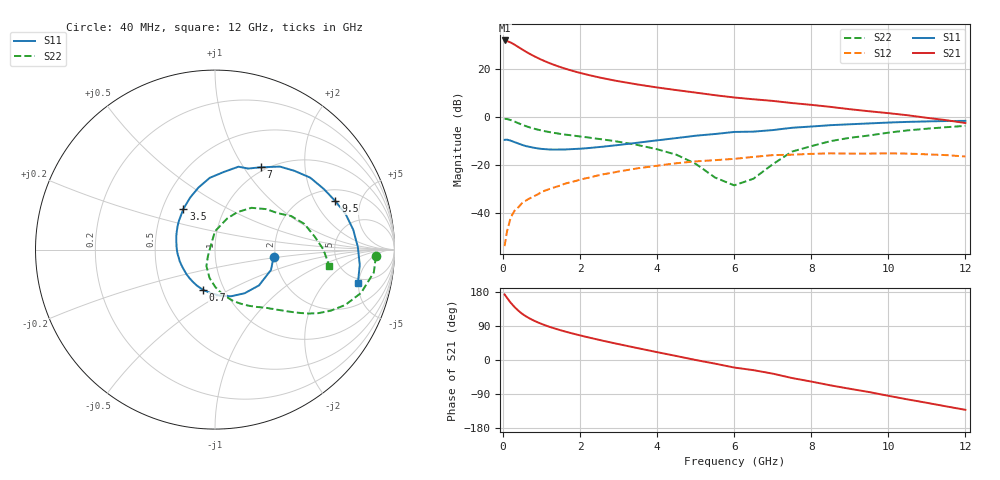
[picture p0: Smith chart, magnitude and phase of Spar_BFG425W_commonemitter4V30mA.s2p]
! Filename: 430bfg425.001
! BFG425W Field C1
! V1=8.371E-001V,V2=4.000E+000V, I1=3.822E-004A, I2=2.995E-002A
# GHz  S  MA  R 50
!  S11  S21  S12  S22
!Freq(GHz)  Mag  Ang  Mag  Ang  Mag  Ang  Mag  Ang
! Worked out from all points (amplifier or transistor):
!   44 points, 40 MHz to 12 GHz, reference 50 ohm
!   highest |S21| = 31.8 dB at 40 MHz (marker M1)
!   |S21| within 3 dB of that: start of sweep to 422.5 MHz
!   unconditionally stable (mu >= 1): start of sweep to 63.48 MHz; 1.129 GHz to end of sweep
!   at 700 MHz: K = 0.86, MSG = 30.0 dB, |S12| = -34.0 dB
!   at 2.4 GHz: K = 1.17, MAG = 18.2 dB, |S12| = -24.7 dB
!   at 12 GHz: K = 1.35, MAG = 3.4 dB, |S12| = -16.6 dB
!   S11 on the Smith chart (normalised r, x): 40 MHz: 1.96, -0.18; 700 MHz: 0.80, -0.38; 3.5 GHz: 0.64, +0.32; 7 GHz: 0.95, +1.20; 9.5 GHz: 2.63, +2.98; 12 GHz: 4.31, -4.89
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0.04  0.329 -7.3  38.74 173.0  0.002 47.2  0.897 -2.3
0.1  0.332 -19.9  37.77 164.5  0.004 70.2  0.894 -8.2
0.2  0.316 -39.1  35.07 150.8  0.008 70.2  0.849 -16.5
0.3  0.294 -55.8  31.55 139.6  0.011 68.4  0.789 -23.0
0.4  0.275 -71.0  28.15 129.9  0.013 66.9  0.729 -27.8
0.5  0.257 -84.7  25.09 121.5  0.016 65.1  0.677 -31.5
0.6  0.243 -96.3  22.44 114.8  0.018 64.0  0.632 -34.3
0.7  0.234 -106.5  20.21 109.1  0.02 63.0  0.594 -36.5
0.9  0.218 -124.5  16.71 99.3  0.024 61.9  0.537 -40.0
1.2  0.207 -145.3  13.11 87.8  0.031 60.2  0.478 -44.4
1.6  0.207 -167.4  10.1 75.5  0.04 57.5  0.425 -49.6
2.2  0.221 167.4  7.448 60.0  0.053 51.8  0.369 -58.3
2.8  0.247 147.4  5.864 46.2  0.067 44.9  0.317 -67.7
3.5  0.287 127.9  4.673 31.2  0.084 35.6  0.256 -79.9
4.5  0.358 104.9  3.577 10.5  0.107 20.8  0.161 -100.9
5.5  0.435 83.6  2.803 -9.6  0.124 5.2  0.054 -137.1
6.5  0.488 67.7  2.304 -26.8  0.145 -7.0  0.051 108.1
7  0.525 60.9  2.132 -36.0  0.158 -14.7  0.102 90.1
8.5  0.665 37.1  1.599 -66.9  0.172 -44.0  0.309 48.9
9.5  0.723 21.9  1.297 -84.6  0.17 -60.7  0.405 30.0
10.5  0.778 8.2  1.069 -104.0  0.17 -79.2  0.518 16.0
12  0.818 -13.3  0.737 -131.4  0.148 -109.2  0.643 -8.0
